| TEXAS INSTRUMENTS INCORPORATED
| High Performance Analog Group
| IBIS Models for output buffers (clock and data) of ADS5500/20/21/22/41/42
| A/D converter
| This file provides unique models under the [Model Selector] keyword for each
| load condition for both clock and data buffers.
| For operation at a specific load condition, select the appropriate model
|after each [Model Selector] keyword.
[IBIS ver]   3.2
[File name]   ads55xx.ibs
[File Rev]   0
[Date]   20 Jan 2005
[Source]   Data created from TI-SPICE simulations
[Disclaimer] Property of
   Texas Instruments Incorporated. Unauthorized reproduction
   protected under copyright law. Created 2005, (C) Copyright
   2005, Texas Instruments Incorporated, All Rights Reserved
   UNLESS THERE IS A SIGNED, WRITTEN AGREEMENT TO THE CONTRARY,
   TEXAS INSTRUMENTS (TI) IS PROVIDING THE IBIS MODELS AND
   WITHOUT ANY WARRANTY, EXPRESSED OR IMPLIED. TI assumes no
   liability for: 1) the accuracy of the IBIS models provided to
   your company; 2) the proper functioning of these IBIS Models
   in your design or for any resulting applications; or 3)
   infringement of patents, copyrights or intellectual property
   rights resulting from your use of these IBIS models. TI
   provides IBIS Models as a service to our customers. You and
   your company shall not distribute, sell or give these models
   to anyone else without prior written permission from TI.
   TI reserves the right to make changes to our products or
   to discontinue any semiconductor product or service
   without notice, and advises our customers to obtain the
   latest version of relevant information to verify, before
   placing orders, that the information being relied on is
   current.
   Please be aware that your receipt and use of the IBIS
   information provided shall serve as acceptance of these
   terms and conditions.  If you do not accept these terms,
   you should return or destroy the IBIS models and any
   other accompanying information immediately.
[Notes]   ADS55XX clock and data output buffers are characterized here
   as 2-state output buffer.
   (In transient simulations use both pairs of V-t curves for
   better results. )
[Copyright]   Property of Texas Instruments Incorporated. Unauthorised
   reproduction and/or distribution is strictly prohibited. This
   product is protected under copyright law and trade secret law
   as an unpublished work. Created 2000,(C) Copyright 2000,Texas
   Instruments Inc., All Rights Reserved.These commodities are
   under the U.S. Government distribution license control.As
   such,they are not to be re-exported without the prior approval
   of the U.S. Department of Commerce.
|   Component ADS55XX
[Component]   ADS55XX
[Manufacturer]   Texas Instruments
[Package]
| variable   typ   min   max
R_pkg   0.019   0.019   0.020
L_pkg   2.580e-9   2.419e-9   2.812e-9
C_pkg   4.82e-13   4.19e-13   5.18e-13
[Pin]   signal_name   model_name   R_pin   L_pin   C_pin
|   (ohms)   (nH)   (pF)
1   DRGND   GND   0.020   2.808e-9   4.20e-13
2   RESERVED   NC   0.019   2.696e-9   5.18e-13
3   RESERVED   NC   0.019   2.634e-9   5.13e-13
4   RESERVED   NC   0.019   2.576e-9   5.02e-13
5   AVDD   POWER   0.019   2.526e-9   4.91e-13
6   AGND   GND   0.019   2.489e-9   4.82e-13
7   AVDD   POWER   0.019   2.473e-9   4.80e-13
8   AGND   GND   0.019   2.419e-9   4.56e-13
9   AVDD   POWER   0.019   2.419e-9   4.56e-13
|10   CLKP   dummy   0.019   2.473e-9   4.80e-13
|11   CLKM   dummy   0.019   2.489e-9   4.82e-13
12   AGND   GND   0.019   2.526e-9   4.91e-13
13   AGND   GND   0.019   2.576e-9   5.02e-13
14   AGND   GND   0.019   2.633e-9   5.13e-13
15   AVDD   POWER   0.019   2.696e-9   5.18e-13
16   AGND   GND   0.020   2.808e-9   4.20e-13
17   CM   POWER   0.020   2.812e-9   4.19e-13
18   AGND   GND   0.019   2.699e-9   5.16e-13
19   INP   NC   0.019   2.638e-9   5.11e-13
20   INM   NC   0.019   2.581e-9   5.00e-13
21   AGND   GND   0.019   2.532e-9   4.88e-13
22   AVDD   POWER   0.019   2.495e-9   4.80e-13
23   AGND   GND   0.019   2.480e-9   4.77e-13
24   AVDD   POWER   0.019   2.427e-9   4.52e-13
25   AGND   GND   0.019   2.427e-9   4.52e-13
26   AVDD   POWER   0.019   2.480e-9   4.77e-13
27   AGND   GND   0.019   2.496e-9   4.80e-13
28   AVDD   POWER   0.019   2.532e-9   4.88e-13
29   REFP   POWER   0.019   2.581e-9   4.99e-13
30   REFM   POWER   0.019   2.638e-9   5.11e-13
|31   IREF   dummy   0.019   2.699e-9   5.17e-13
32   AGND   GND   0.020   2.811e-9   4.19e-13
33   AVDD   POWER   0.020   2.809e-9   4.20e-13
34   AVDD   POWER   0.019   2.698e-9   5.18e-13
|35   RESET   dummy   0.019   2.637e-9   5.13e-13
36   AGND   GND   0.019   2.579e-9   5.02e-13
37   AVDD   POWER   0.019   2.529e-9   4.91e-13
38   AGND   GND   0.019   2.492e-9   4.83e-13
39   AVDD   POWER   0.019   2.476e-9   4.80e-13
|40   DFS   dummy   0.019   2.422e-9   4.57e-13
|41   OE   dummy   0.019   2.422e-9   4.57e-13
42   DRGND   GND   0.019   2.476e-9   4.80e-13
43   CLKOUT   CLKOBUF   0.019   2.492e-9   4.83e-13
44   D0   DATAOBUF   0.019   2.530e-9   4.91e-13
45   D1   DATAOBUF   0.019   2.579e-9   5.02e-13
46   D2   DATAOBUF   0.019   2.637e-9   5.13e-13
47   D3   DATAOBUF   0.019   2.698e-9   5.18e-13
48   DRGND   GND   0.020   2.809e-9   4.20e-13
49   DRVDD   POWER   0.020   2.809e-9   4.19e-13
50   DRGND   GND   0.019   2.695e-9   5.17e-13
51   D4   DATAOBUF   0.019   2.633e-9   5.12e-13
52   D5   DATAOBUF   0.019   2.576e-9   5.01e-13
53   D6   DATAOBUF   0.019   2.526e-9   4.90e-13
54   D7   DATAOBUF   0.019   2.489e-9   4.81e-13
55   D8   DATAOBUF   0.019   2.474e-9   4.78e-13
56   D9   DATAOBUF   0.019   2.421e-9   4.53e-13
57   DRGND   GND   0.019   2.421e-9   4.53e-13
58   DRVDD   POWER   0.019   2.474e-9   4.78e-13
59   DRGND   GND   0.019   2.490e-9   4.81e-13
60   D10   DATAOBUF   0.019   2.526e-9   4.89e-13
61   D11   DATAOBUF   0.019   2.576e-9   5.01e-13
62   D12   DATAOBUF   0.019   2.633e-9   5.12e-13
63   D13   DATAOBUF   0.019   2.695e-9   5.17e-13
64   OVR   DATAOBUF   0.020   2.809e-9   4.19e-13
[Model Selector] DATAOBUF
| Each model described below models the data buffer operating at a particular
| speed, driving a particular transmission line, terminated by a particular
| load capacitor.
| Syntax for naming model is:
| DATAOBUF_<speed>_<transmisson line delay>_<terminating capacitor>
| Following 2 examples illustrate this notation.
| (1) DATAOBUF_125_0_4 is the model of buffer operating at 125MSPS,
| driving a 4 pF capacitive load with no transmission line.
| (2) DATAOBUF_80_400_12 is the model of buffer operating at 80MSPS,
|driving a transmission line of delay 400ps and terminated by capacitor of 12pF
|  Model name   speed   delay line   capacitive_load
DATAOBUF_125_0_4   125 MSPS   no delay line   4  pF
DATAOBUF_125_0_8   125 MSPS   no delay line   8  pF
DATAOBUF_125_0_12   125 MSPS   no delay line   12 pF
DATAOBUF_125_0_15   125 MSPS   no delay line   15 pF
DATAOBUF_125_400_4   125 MSPS   400 ps delay line   4  pF
DATAOBUF_125_400_8   125 MSPS   400 ps delay line   8  pF
DATAOBUF_125_400_12   125 MSPS   400 ps delay line   12 pF
DATAOBUF_125_400_15   125 MSPS   400 ps delay line   15 pF
DATAOBUF_125_600_4   125 MSPS   600 ps delay line   4  pF
DATAOBUF_125_600_8   125 MSPS   600 ps delay line   8  pF
DATAOBUF_125_600_12   125 MSPS   600 ps delay line   12 pF
DATAOBUF_125_600_15   125 MSPS   600 ps delay line   15 pF
DATAOBUF_125_800_4   125 MSPS   800 ps delay line   4  pF
DATAOBUF_125_800_8   125 MSPS   800 ps delay line   8  pF
DATAOBUF_125_800_12   125 MSPS   800 ps delay line   12 pF
DATAOBUF_125_800_15   125 MSPS   800 ps delay line   15 pF
DATAOBUF_105_0_4   105 MSPS   no delay line   4  pF
DATAOBUF_105_0_8   105 MSPS   no delay line   8  pF
DATAOBUF_105_0_12   105 MSPS   no delay line   12 pF
DATAOBUF_105_0_15   105 MSPS   no delay line   15 pF
DATAOBUF_105_400_4   105 MSPS   400 ps delay line   4  pF
DATAOBUF_105_400_8   105 MSPS   400 ps delay line   8  pF
DATAOBUF_105_400_12   105 MSPS   400 ps delay line   12 pF
DATAOBUF_105_400_15   105 MSPS   400 ps delay line   15 pF
DATAOBUF_105_600_4   105 MSPS   600 ps delay line   4  pF
DATAOBUF_105_600_8   105 MSPS   600 ps delay line   8  pF
DATAOBUF_105_600_12   105 MSPS   600 ps delay line   12 pF
DATAOBUF_105_600_15   105 MSPS   600 ps delay line   15 pF
DATAOBUF_105_800_4   105 MSPS   800 ps delay line   4  pF
DATAOBUF_105_800_8   105 MSPS   800 ps delay line   8  pF
DATAOBUF_105_800_12   105 MSPS   800 ps delay line   12 pF
DATAOBUF_105_800_15   105 MSPS   800 ps delay line   15 pF
DATAOBUF_80_0_4   80  MSPS   no delay line   4  pF
DATAOBUF_80_0_8   80  MSPS   no delay line   8  pF
DATAOBUF_80_0_12   80  MSPS   no delay line   12 pF
DATAOBUF_80_0_15   80  MSPS   no delay line   15 pF
DATAOBUF_80_400_4   80  MSPS   400 ps delay line   4  pF
DATAOBUF_80_400_8   80  MSPS   400 ps delay line   8  pF
DATAOBUF_80_400_12   80  MSPS   400 ps delay line   12 pF
DATAOBUF_80_400_15   80  MSPS   400 ps delay line   15 pF
DATAOBUF_80_600_4   80  MSPS   600 ps delay line   4  pF
DATAOBUF_80_600_8   80  MSPS   600 ps delay line   8  pF
DATAOBUF_80_600_12   80  MSPS   600 ps delay line   12 pF
DATAOBUF_80_600_15   80  MSPS   600 ps delay line   15 pF
DATAOBUF_80_800_4   80  MSPS   800 ps delay line   4  pF
DATAOBUF_80_800_8   80  MSPS   800 ps delay line   8  pF
DATAOBUF_80_800_12   80  MSPS   800 ps delay line   12 pF
DATAOBUF_80_800_15   80  MSPS   800 ps delay line   15 pF
[Model Selector] CLKOBUF
| Each model described below models the buffer operating at a particular speed,
| driving a particular load, terminated by a particular load capacitor.
| Syntax for naming model is:
|CLKOBUF_<speed>_<transmisson line delay>_<terminating capacitor>
| Following 2 examples illustrate this notation.
| (1) CLKOBUF_125_0_4 is the model of buffer operating at 125MSPS,
| driving a 4 pF capacitive load with no transmission line.
| (2) CLKOBUF_80_400_12 is the model of buffer operating at 80MSPS,
|driving a transmission line of delay 400ps and terminated by capacitor of 12pF
|  Model name   speed   delay line   capacitive_load
CLKOBUF_125_0_4   125 MSPS   no delay line   4  pF
CLKOBUF_125_0_8   125 MSPS   no delay line   8  pF
CLKOBUF_125_0_12   125 MSPS   no delay line   12 pF
CLKOBUF_125_0_15   125 MSPS   no delay line   15 pF
CLKOBUF_125_400_4   125 MSPS   400 ps delay line   4  pF
CLKOBUF_125_400_8   125 MSPS   400 ps delay line   8  pF
CLKOBUF_125_400_12   125 MSPS   400 ps delay line   12 pF
CLKOBUF_125_400_15   125 MSPS   400 ps delay line   15 pF
CLKOBUF_125_600_4   125 MSPS   600 ps delay line   4  pF
CLKOBUF_125_600_8   125 MSPS   600 ps delay line   8  pF
CLKOBUF_125_600_12   125 MSPS   600 ps delay line   12 pF
CLKOBUF_125_600_15   125 MSPS   600 ps delay line   15 pF
CLKOBUF_125_800_4   125 MSPS   800 ps delay line   4  pF
CLKOBUF_125_800_8   125 MSPS   800 ps delay line   8  pF
CLKOBUF_125_800_12   125 MSPS   800 ps delay line   12 pF
CLKOBUF_125_800_15   125 MSPS   800 ps delay line   15 pF
CLKOBUF_105_0_4   105 MSPS   no delay line   4  pF
CLKOBUF_105_0_8   105 MSPS   no delay line   8  pF
CLKOBUF_105_0_12   105 MSPS   no delay line   12 pF
CLKOBUF_105_0_15   105 MSPS   no delay line   15 pF
CLKOBUF_105_400_4   105 MSPS   400 ps delay line   4  pF
CLKOBUF_105_400_8   105 MSPS   400 ps delay line   8  pF
CLKOBUF_105_400_12   105 MSPS   400 ps delay line   12 pF
CLKOBUF_105_400_15   105 MSPS   400 ps delay line   15 pF
CLKOBUF_105_600_4   105 MSPS   600 ps delay line   4  pF
CLKOBUF_105_600_8   105 MSPS   600 ps delay line   8  pF
CLKOBUF_105_600_12   105 MSPS   600 ps delay line   12 pF
CLKOBUF_105_600_15   105 MSPS   600 ps delay line   15 pF
CLKOBUF_105_800_4   105 MSPS   800 ps delay line   4  pF
CLKOBUF_105_800_8   105 MSPS   800 ps delay line   8  pF
CLKOBUF_105_800_12   105 MSPS   800 ps delay line   12 pF
CLKOBUF_105_800_15   105 MSPS   800 ps delay line   15 pF
CLKOBUF_80_0_4   80  MSPS   no delay line   4  pF
CLKOBUF_80_0_8   80  MSPS   no delay line   8  pF
CLKOBUF_80_0_12   80  MSPS   no delay line   12 pF
CLKOBUF_80_0_15   80  MSPS   no delay line   15 pF
CLKOBUF_80_400_4   80  MSPS   400 ps delay line   4  pF
CLKOBUF_80_400_8   80  MSPS   400 ps delay line   8  pF
CLKOBUF_80_400_12   80  MSPS   400 ps delay line   12 pF
CLKOBUF_80_400_15   80  MSPS   400 ps delay line   15 pF
CLKOBUF_80_600_4   80  MSPS   600 ps delay line   4  pF
CLKOBUF_80_600_8   80  MSPS   600 ps delay line   8  pF
CLKOBUF_80_600_12   80  MSPS   600 ps delay line   12 pF
CLKOBUF_80_600_15   80  MSPS   600 ps delay line   15 pF
CLKOBUF_80_800_4   80  MSPS   800 ps delay line   4  pF
CLKOBUF_80_800_8   80  MSPS   800 ps delay line   8  pF
CLKOBUF_80_800_12   80  MSPS   800 ps delay line   12 pF
CLKOBUF_80_800_15   80  MSPS   800 ps delay line   15 pF
| Models and submodels in the file (96): DATAOBUF_125_0_4 (Output), DATAOBUF_125_0_8 (Output), DATAOBUF_125_0_12 (Output), DATAOBUF_125_0_15 (Output), DATAOBUF_125_400_4 (Output), DATAOBUF_125_400_8 (Output), DATAOBUF_125_400_12 (Output), DATAOBUF_125_400_15 (Output), DATAOBUF_125_600_4 (Output), DATAOBUF_125_600_8 (Output), DATAOBUF_125_600_12 (Output), DATAOBUF_125_600_15 (Output), DATAOBUF_125_800_4 (Output), DATAOBUF_125_800_8 (Output), DATAOBUF_125_800_12 (Output), DATAOBUF_125_800_15 (Output), DATAOBUF_105_0_4 (Output), DATAOBUF_105_0_8 (Output), DATAOBUF_105_0_12 (Output), DATAOBUF_105_0_15 (Output), DATAOBUF_105_400_4 (Output), DATAOBUF_105_400_8 (Output), DATAOBUF_105_400_12 (Output), DATAOBUF_105_400_15 (Output), DATAOBUF_105_600_4 (Output), DATAOBUF_105_600_8 (Output), DATAOBUF_105_600_12 (Output), DATAOBUF_105_600_15 (Output), DATAOBUF_105_800_4 (Output), DATAOBUF_105_800_8 (Output), DATAOBUF_105_800_12 (Output), DATAOBUF_105_800_15 (Output), DATAOBUF_80_0_4 (Output), DATAOBUF_80_0_8 (Output), DATAOBUF_80_0_12 (Output), DATAOBUF_80_0_15 (Output), DATAOBUF_80_400_4 (Output), DATAOBUF_80_400_8 (Output), DATAOBUF_80_400_12 (Output), DATAOBUF_80_400_15 (Output), DATAOBUF_80_600_4 (Output), DATAOBUF_80_600_8 (Output), DATAOBUF_80_600_12 (Output), DATAOBUF_80_600_15 (Output), DATAOBUF_80_800_4 (Output), DATAOBUF_80_800_8 (Output), DATAOBUF_80_800_12 (Output), DATAOBUF_80_800_15 (Output), CLKOBUF_125_0_4 (Output), CLKOBUF_125_0_8 (Output), CLKOBUF_125_0_12 (Output), CLKOBUF_125_0_15 (Output), CLKOBUF_125_400_4 (Output), CLKOBUF_125_400_8 (Output), CLKOBUF_125_400_12 (Output), CLKOBUF_125_400_15 (Output), CLKOBUF_125_600_4 (Output), CLKOBUF_125_600_8 (Output), CLKOBUF_125_600_12 (Output), CLKOBUF_125_600_15 (Output), CLKOBUF_125_800_4 (Output), CLKOBUF_125_800_8 (Output), CLKOBUF_125_800_12 (Output), CLKOBUF_125_800_15 (Output), CLKOBUF_105_0_4 (Output), CLKOBUF_105_0_8 (Output), CLKOBUF_105_0_12 (Output), CLKOBUF_105_0_15 (Output), CLKOBUF_105_400_4 (Output), CLKOBUF_105_400_8 (Output), CLKOBUF_105_400_12 (Output), CLKOBUF_105_400_15 (Output), CLKOBUF_105_600_4 (Output), CLKOBUF_105_600_8 (Output), CLKOBUF_105_600_12 (Output), CLKOBUF_105_600_15 (Output), CLKOBUF_105_800_4 (Output), CLKOBUF_105_800_8 (Output), CLKOBUF_105_800_12 (Output), CLKOBUF_105_800_15 (Output)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
